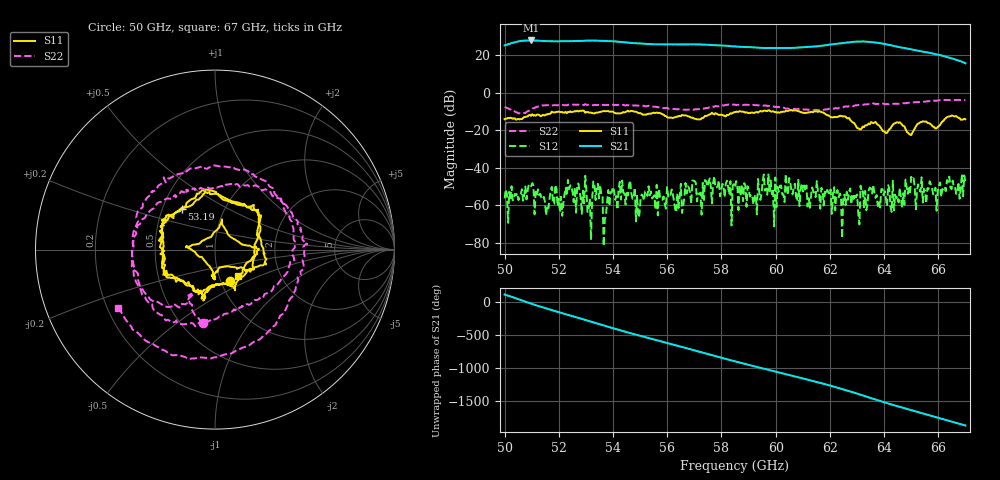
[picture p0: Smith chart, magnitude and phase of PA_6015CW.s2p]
!Agilent Technologies,E8361A,US42410132,A.06.03.05
!Agilent E8361A: A.06.03.05
!Date: Friday, July 11, 2008 12:57:41
!Correction: S11(Full 2 Port(1,2)) S21(Full 2 Port(1,2)) S12(Full 2 Port(1,2)) S22(Full 2 Port(1,2))
!S2P File: Measurements: S11, S21, S12, S22:
# Hz S  MA  R 50
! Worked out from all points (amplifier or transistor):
!   401 points, 50 GHz to 67 GHz, reference 50 ohm
!   highest |S21| = 27.7 dB at 50.98 GHz (marker M1)
!   |S21| within 3 dB of that: start of sweep to 58.3 GHz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
!   unconditionally stable (mu >= 1): start of sweep to end of sweep
!   at 52.8 GHz: K = 9.18, MAG = 29.0 dB, |S12| = -55.9 dB
!   at 58.5 GHz: K = 7.00, MAG = 25.9 dB, |S12| = -50.3 dB
!   at 67 GHz: K = 11.29, MAG = 17.9 dB, |S12| = -47.4 dB
!   S11 on the Smith chart (normalised r, x): 50 GHz: 1.10, -0.41; 53.19 GHz: 0.63, +0.31; 67 GHz: 1.23, -0.38
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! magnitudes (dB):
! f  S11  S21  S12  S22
! 50 GHz  -14.2  25.1  -56.2  -7.7
! 50.98 GHz  -12.4  27.7  -49.8  -8.9
! 51.53 GHz  -11.7  27.3  -65.2  -6.7
! 52.42 GHz  -10.0  27.3  -49.3  -6.4
! 52.85 GHz  -9.7  27.4  -64.4  -6.5
! 53.19 GHz  -10.7  27.6  -78.3  -6.7
! 53.36 GHz  -10.8  27.6  -57.1  -6.6
! 53.7 GHz  -9.9  27.4  -67.3  -6.7
! 53.91 GHz  -10.2  27.3  -52.9  -6.7
! 54.29 GHz  -11.1  26.9  -56.9  -6.6
! 54.93 GHz  -10.8  26.1  -66.3  -7.0
! 55.7 GHz  -10.8  25.6  -51.2  -7.8
! 58.5 GHz  -10.4  24.5  -50.3  -6.5
! 59.22 GHz  -10.7  23.9  -55.2  -6.7
! 59.65 GHz  -9.7  23.7  -50.9  -6.9
! 59.95 GHz  -10.2  23.7  -71.1  -7.5
! 60.45 GHz  -9.8  23.7  -54.5  -8.5
! 61.35 GHz  -10.4  24.3  -50.4  -9.3
! 64.19 GHz  -19.5  25.3  -51.2  -6.1
! 65.05 GHz  -21.2  22.8  -46.2  -5.3
! 65.89 GHz  -19.1  20.5  -50.5  -4.4
! 67 GHz  -14.2  15.5  -47.4  -4.0
